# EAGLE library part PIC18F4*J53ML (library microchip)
PIC18F47J53 Family High-Performance USB Microcontrollers with nanoWatt XLP Technology Source: Data sheet
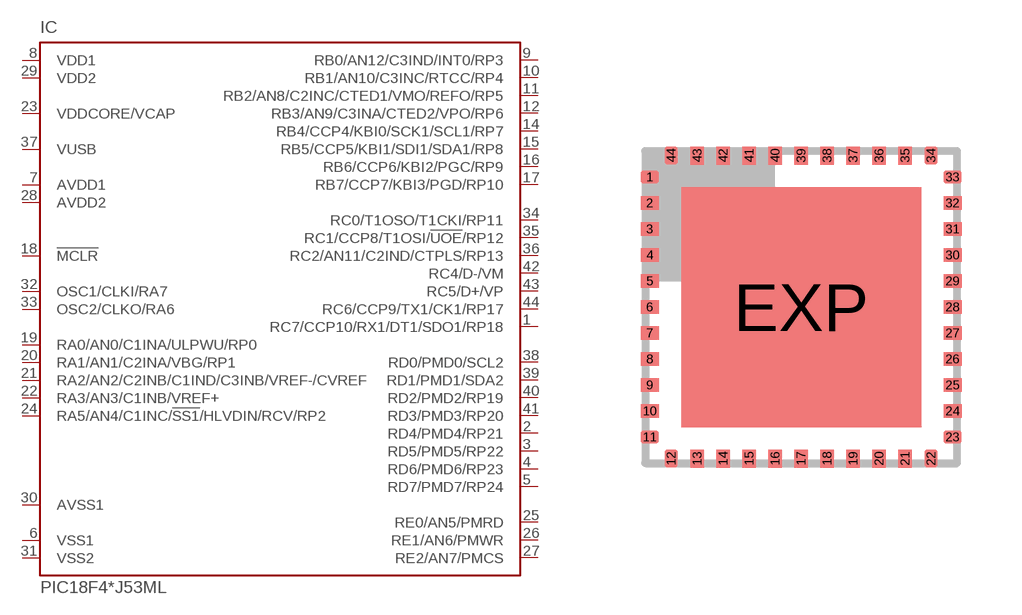
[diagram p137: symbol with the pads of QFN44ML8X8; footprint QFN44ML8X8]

Designator prefix IC

## PIC18F46J53ML (MPN: PIC18F46J53-I/ML; OC_FARNELL: unknown; OC_NEWARK: 63R7851), PIC18F47J53ML (MPN: PIC18F47J53-I/ML; OC_FARNELL: 1815000; OC_NEWARK: 63R7855)  [QFN44ML8X8]
1  RC7/CCP10/RX1/DT1/SDO1/RP18
2  RD4/PMD4/RP21
3  RD5/PMD5/RP22
4  RD6/PMD6/RP23
5  RD7/PMD7/RP24
6  VSS1  in
7  AVDD1  in
8  VDD1  in
9  RB0/AN12/C3IND/INT0/RP3
10  RB1/AN10/C3INC/RTCC/RP4
11  RB2/AN8/C2INC/CTED1/VMO/REFO/RP5
12  RB3/AN9/C3INA/CTED2/VPO/RP6
14  RB4/CCP4/KBI0/SCK1/SCL1/RP7
15  RB5/CCP5/KBI1/SDI1/SDA1/RP8
16  RB6/CCP6/KBI2/PGC/RP9
17  RB7/CCP7/KBI3/PGD/RP10
18  !MCLR  in
19  RA0/AN0/C1INA/ULPWU/RP0
20  RA1/AN1/C2INA/VBG/RP1
21  RA2/AN2/C2INB/C1IND/C3INB/VREF-/CVREF
22  RA3/AN3/C1INB/VREF+
23  VDDCORE/VCAP  in
24  RA5/AN4/C1INC/!SS1!/HLVDIN/RCV/RP2
25  RE0/AN5/PMRD
26  RE1/AN6/PMWR
27  RE2/AN7/PMCS
28  AVDD2  in
29  VDD2  in
30  AVSS1  in
31  VSS2  in
32  OSC1/CLKI/RA7
33  OSC2/CLKO/RA6
34  RC0/T1OSO/T1CKI/RP11
35  RC1/CCP8/T1OSI/!UOE!/RP12
36  RC2/AN11/C2IND/CTPLS/RP13
37  VUSB  in
38  RD0/PMD0/SCL2
39  RD1/PMD1/SDA2
40  RD2/PMD2/RP19
41  RD3/PMD3/RP20
42  RC4/D-/VM
43  RC5/D+/VP
44  RC6/CCP9/TX1/CK1/RP17

## Footprint QFN44ML8X8 (pad centres in mm)
44-Lead Plastic Quad Flat No Lead Package (ML) 8x8 mm Body (QFN) Source: http://ww1.microchip.com/downloads/en/devicedoc/39632c.pdf
smd 0.45 x 0.33: 1 -3.788,3.25; 2 -3.788,2.6; 3 -3.788,1.95; 4 -3.788,1.3; 5 -3.788,0.65; 6 -3.788,0; 7 -3.788,-0.65; 8 -3.788,-1.3; 9 -3.788,-1.95; 10 -3.788,-2.6; 11 -3.788,-3.25; 23 3.788,-3.25; 24 3.788,-2.6; 25 3.788,-1.95; 26 3.788,-1.3; 27 3.788,-0.65; 28 3.788,0; 29 3.788,0.65; 30 3.788,1.3; 31 3.788,1.95; 32 3.788,2.6; 33 3.788,3.25
smd 0.33 x 0.45: 12 -3.25,-3.788; 13 -2.6,-3.788; 14 -1.95,-3.788; 15 -1.3,-3.788; 16 -0.65,-3.788; 17 0,-3.788; 18 0.65,-3.788; 19 1.3,-3.788; 20 1.95,-3.788; 21 2.6,-3.788; 22 3.25,-3.788; 34 3.25,3.788; 35 2.6,3.788; 36 1.95,3.788; 37 1.3,3.788; 38 0.65,3.788; 39 0,3.788; 40 -0.65,3.788; 41 -1.3,3.788; 42 -1.95,3.788; 43 -2.6,3.788; 44 -3.25,3.788
smd 6 x 6: EXP 0,0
